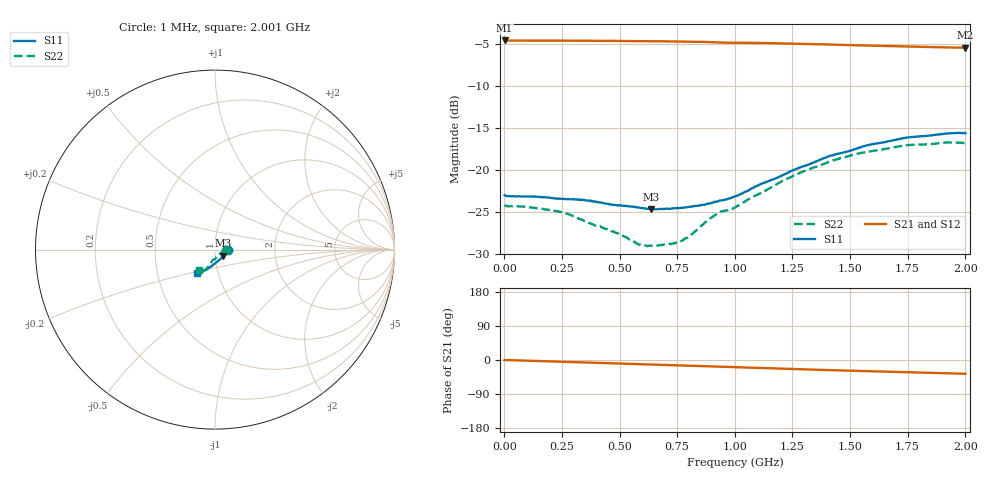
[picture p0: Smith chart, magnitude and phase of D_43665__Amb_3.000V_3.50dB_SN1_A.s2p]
! device id: 43665_
! dir: \\malibu\benchdata\1_engineers\tn_data\43665_75ohm\new\sparar\43665_\amb\3p000v\3p50db
! Serial: 1
! Insertion: A
! Temp: Amb
! VDD: 3.000V
! Attenuation Step: 3.50dB
! IDD: 1.451226e+00mA
! FILE NAME
! DATE 03-27-2009 08:34:14
! CORRECTED  DATA
#  Hz  S  RI  R  75
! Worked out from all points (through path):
!   401 points, 1 MHz to 2.001 GHz, reference 75 ohm
!   highest |S21| = -4.54 dB at 1 MHz (marker M1); lowest = -5.4 dB at 2.001 GHz (marker M2)
!   group delay of S21, straight-line fit = 51.4 ps
!   lowest |S11| = -24.7 dB at 636 MHz (marker M3), VSWR 1.12, Z = 82.2 - j5.72 ohm
!   |S11| at or under -10 dB: start of sweep to end of sweep
!   |S22| runs from -29.1 to -16.7 dB; largest |S21 - S12| = 0.0029
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1000000  0.071 -0.00102  0.5928 -0.000907  0.593 -0.0011  0.062 -0.000891
2.21e8  0.0673 -0.0081  0.5898 -0.0419  0.59 -0.0422  0.057 -0.00344
2.76e8  0.0663 -0.0113  0.5887 -0.0525  0.5889 -0.0527  0.0547 -0.00384
3.36e8  0.0652 -0.0142  0.587 -0.064  0.5872 -0.0642  0.0504 -0.00539
4.81e8  0.0578 -0.0225  0.5819 -0.0918  0.582 -0.0921  0.0404 -0.013
5.81e8  0.0517 -0.0305  0.5766 -0.1108  0.5767 -0.1111  0.0309 -0.019
6.36e8  0.047 -0.0347  0.5739 -0.1211  0.5738 -0.1214  0.0265 -0.0234
6.71e8  0.0445 -0.0382  0.572 -0.1278  0.5719 -0.128  0.0239 -0.0265
7.31e8  0.0399 -0.0438  0.5682 -0.1394  0.5682 -0.1395  0.0185 -0.0315
7.71e8  0.036 -0.0476  0.5652 -0.1472  0.5651 -0.1473  0.0138 -0.0354
8.06e8  0.0326 -0.0511  0.5624 -0.1541  0.5623 -0.1542  0.0102 -0.0395
9.21e8  0.0175 -0.0625  0.55 -0.1753  0.5502 -0.1752  -0.00299 -0.0547
1.001e9  0.00964 -0.069  0.5437 -0.1857  0.544 -0.1858  -0.014 -0.0582
1.211e9  -0.0196 -0.0916  0.5241 -0.2221  0.5248 -0.2224  -0.0279 -0.0822
1.336e9  -0.037 -0.1039  0.5097 -0.2404  0.5104 -0.2409  -0.0387 -0.0954
1.406e9  -0.0474 -0.111  0.5013 -0.2511  0.5021 -0.2521  -0.0427 -0.1033
1.521e9  -0.0625 -0.1179  0.4876 -0.2654  0.4881 -0.2667  -0.0543 -0.1117
1.581e9  -0.0698 -0.1231  0.4805 -0.2732  0.4809 -0.2749  -0.0575 -0.1154
1.671e9  -0.0788 -0.1265  0.47 -0.2836  0.4694 -0.2852  -0.0652 -0.1185
1.746e9  -0.0861 -0.1305  0.461 -0.2919  0.4606 -0.2938  -0.0707 -0.1218
1.916e9  -0.0971 -0.1335  0.4416 -0.3092  0.4405 -0.3097  -0.0832 -0.1201
2.001e9  -0.0995 -0.133  0.4323 -0.3174  0.4297 -0.3189  -0.0865 -0.1163
